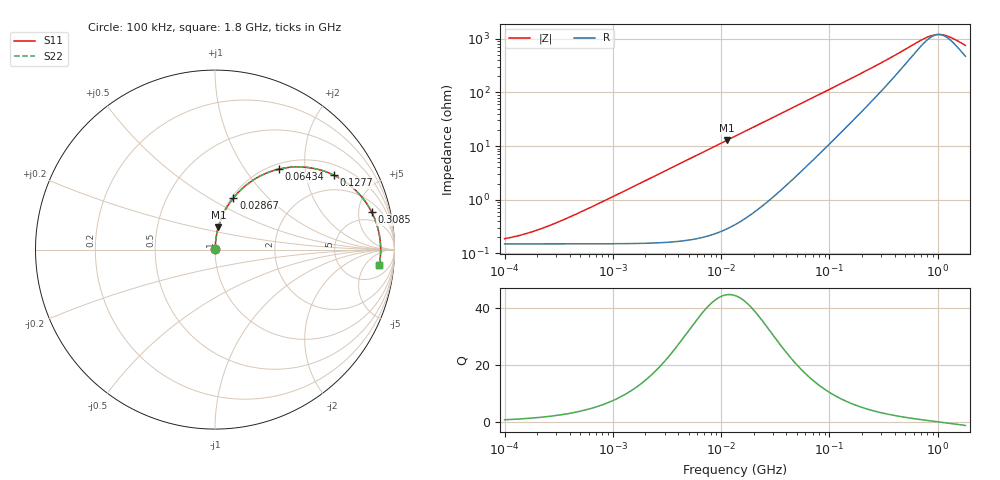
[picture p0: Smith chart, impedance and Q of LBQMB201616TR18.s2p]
! LBQMB201616TR18  S-PARAMETER MODEL  ( General Type )
! Model Generated by TAIYO YUDEN Corporation (http://www.ty-top.com)
! Version 1.0
! TAIYO YUDEN Control No. 191025NI43SB-FBB
! Copyright(c) 2019 TAIYO YUDEN CO.,LTD. All Rights Reserved.
! Product Description (link to TY-COMPAS)
! https://ds.yuden.co.jp/TYCOMPAS/or/detail?pn=LBQMB201616TR18J&u=M
! Products Name : Inductors
! Characteristics :
!  Inductance : 0.18 uH , SRF(min) : 500 MHz , DC Resistance(max) : 0.195 Ohm , Rated Current : 560 mA
!  Case Size : 2.0 x 1.6 / 0.079 x 0.063 [mm/inch] , Thickness : 1.6 / 0.063 [mm/inch]
!  (Conditions: Temperature = 25 degC , DC Bias Current/Voltage = 0A / 0V)
! External Node Assignments :
!  1  o---GGG---o  2
! GND o---------o GND
! Frequency Range : 0.1MHz  -  1800MHz  [ 402 STEP ]
# MHz S RI R 50
! Freq[MHz].  S11 Real  S11 Imag  S21 Real  S21 Imag  S12 Real  S12 Imag  S22 Real  S22 Imag
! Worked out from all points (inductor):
!   401 points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, 100 kHz to 1.8 GHz, reference 50 ohm
!   read as one part in series: L = 180 nH near 404 kHz
!   highest Q = 44.7 at 11.3 MHz (marker M1), where L = 180 nH
!   self-resonance near 1.021 GHz
!   S11 on the Smith chart (normalised r, x): 100 kHz: 1.00, +0.00; 28.67 MHz: 1.02, +0.65; 64.34 MHz: 1.09, +1.46; 127.7 MHz: 1.36, +2.89; 308.5 MHz: 3.23, +6.97; 1.8 GHz: 10, -12
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0.1  0.0015 0.00113  0.9985 -0.00113  0.9985 -0.00113  0.0015 0.00113
0.140908  0.0015 0.00159  0.9985 -0.00159  0.9985 -0.00159  0.0015 0.00159
0.208519  0.0015 0.00235  0.9985 -0.00235  0.9985 -0.00235  0.0015 0.00235
0.516129  0.00153 0.00582  0.9985 -0.00582  0.9985 -0.00582  0.00153 0.00582
2.66389  0.00248 0.03  0.9975 -0.03  0.9975 -0.03  0.00248 0.03
5.97828  0.0064 0.0671  0.9936 -0.0671  0.9936 -0.0671  0.0064 0.0671
11.30236  0.0188 0.1251  0.9812 -0.1251  0.9812 -0.1251  0.0188 0.1251
13.41641  0.0257 0.1473  0.9743 -0.1473  0.9743 -0.1473  0.0257 0.1473
28.66948  0.1026 0.288  0.8974 -0.288  0.8974 -0.288  0.1026 0.288
42.42587  0.1976 0.3772  0.8024 -0.3772  0.8024 -0.3772  0.1976 0.3772
64.33982  0.3558 0.4483  0.6442 -0.4483  0.6442 -0.4483  0.3558 0.4483
69.24595  0.3887 0.4549  0.6113 -0.4549  0.6113 -0.4549  0.3887 0.4549
92.90788  0.5248 0.4565  0.4752 -0.4565  0.4752 -0.4565  0.5248 0.4565
127.7465  0.6614 0.4156  0.3386 -0.4156  0.3386 -0.4156  0.6614 0.4156
193.7305  0.7923 0.3216  0.2077 -0.3216  0.2077 -0.3216  0.7923 0.3216
308.5485  0.8726 0.2097  0.1274 -0.2097  0.1274 -0.2097  0.8726 0.2097
357.3983  0.8874 0.1778  0.1126 -0.1778  0.1126 -0.1778  0.8874 0.1778
727.2099  0.9203 0.0508  0.0797 -0.0508  0.0797 -0.0508  0.9203 0.0508
929.0554  0.9229 0.0139  0.0771 -0.0139  0.0771 -0.0139  0.9229 0.0139
1050.104  0.9231 -0.0042  0.0769 0.0042  0.0769 0.0042  0.9231 -0.0042
1216.359  0.9224 -0.026  0.0776 0.026  0.0776 0.026  0.9224 -0.026
1800  0.9147 -0.0875  0.0853 0.0875  0.0853 0.0875  0.9147 -0.0875
